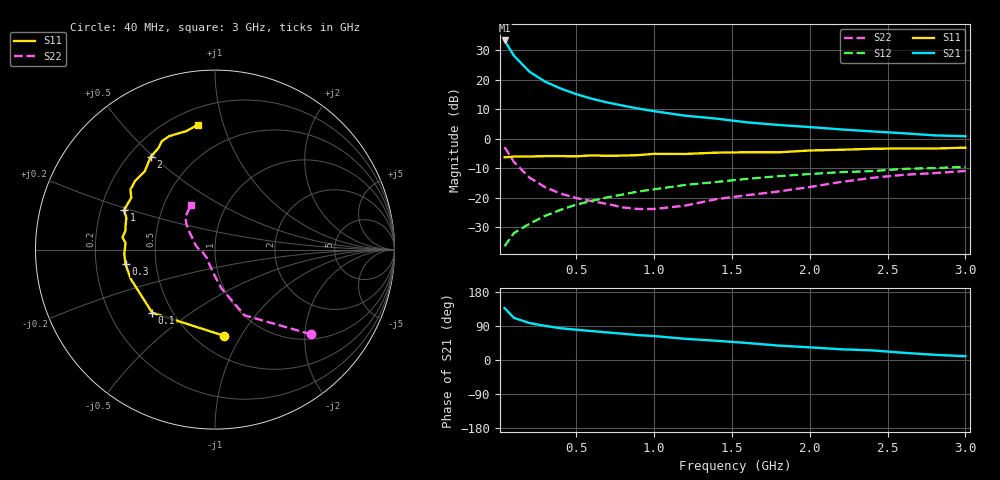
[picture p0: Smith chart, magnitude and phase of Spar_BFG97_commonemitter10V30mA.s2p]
! Filename:  BFG97F.S2P  Version:  2.0
! NXP part #: BFG97  Date: Jul 1990
! Bias condition: Vce=10V, Ic=30mA
#  MHz  S  MA  R  50
! Freq  S11  S21  S12  S22  !GUM [dB]
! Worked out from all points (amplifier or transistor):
!   21 points, 40 MHz to 3 GHz, reference 50 ohm
!   highest |S21| = 33.3 dB at 40 MHz (marker M1)
!   |S21| within 3 dB of that: start of sweep to 74.7 MHz
!   unconditionally stable (mu >= 1): 328.5 MHz to end of sweep
!   at 300 MHz: K = 0.99, MSG = 22.8 dB, |S12| = -26.2 dB
!   at 1 GHz: K = 1.08, MAG = 11.5 dB, |S12| = -17.2 dB
!   at 3 GHz: K = 1.01, MAG = 4.4 dB, |S12| = -9.6 dB
!   S11 on the Smith chart (normalised r, x): 40 MHz: 0.68, -0.85; 100 MHz: 0.39, -0.36; 300 MHz: 0.33, -0.07; 1 GHz: 0.30, +0.19; 2 GHz: 0.29, +0.49; 3 GHz: 0.30, +0.83
40  0.482 -84.2  46.2 136.9  0.015 61.3  0.714 -41.4
100  0.496 -134.8  25.43 111.1  0.025 55.6  0.401 -65.8
200  0.497 -160.7  13.62 97.5  0.036 61.5  0.218 -80.8
300  0.505 -170.8  9.259 90.0  0.049 65.3  0.15 -89.7
400  0.506 -177.4  7.066 83.8  0.062 65.4  0.117 -97.8
500  0.5 175.7  5.681 79.9  0.076 68.1  0.098 -104.8
600  0.52 172.5  4.743 76.3  0.088 67.0  0.087 -111.6
700  0.51 168.0  4.094 72.8  0.101 67.3  0.078 -119.5
800  0.516 164.9  3.627 69.3  0.113 66.3  0.068 -127.1
900  0.525 160.2  3.229 65.6  0.127 66.1  0.064 -137.6
1000  0.552 156.6  2.918 63.2  0.138 64.3  0.064 -147.5
1200  0.549 148.2  2.447 55.9  0.164 62.6  0.073 -172.6
1400  0.578 144.6  2.184 50.8  0.184 60.3  0.094 176.1
1600  0.587 139.3  1.883 44.8  0.208 58.4  0.11 167.5
1800  0.586 131.9  1.704 38.0  0.231 54.0  0.127 159.2
2000  0.629 124.7  1.57 33.4  0.251 52.3  0.151 150.3
2200  0.647 119.2  1.433 28.3  0.27 49.7  0.184 143.4
2400  0.672 116.3  1.324 25.4  0.281 49.0  0.216 137.9
2600  0.682 112.0  1.233 19.1  0.307 44.9  0.243 132.5
2800  0.679 103.6  1.136 13.8  0.316 40.5  0.26 125.9
3000  0.703 97.7  1.096 9.9  0.332 39.1  0.283 117.8
